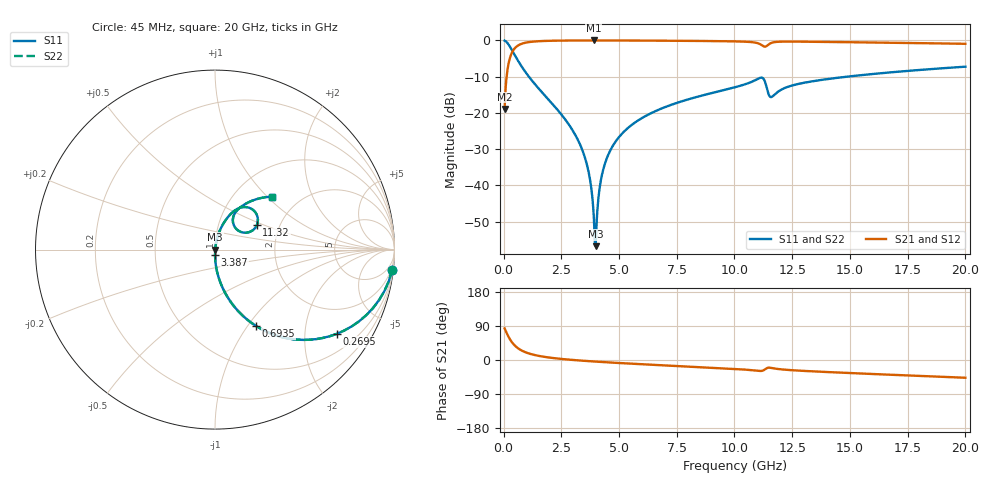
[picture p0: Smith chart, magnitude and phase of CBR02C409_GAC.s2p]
! S-parameter model data by Modelithics Inc.  support@modelithics.com 813-866-6335  Tampa FL USA
! S-Parameter data specifications:
! Substrate: 20-mil Rogers 4350B, substrate thickness, H=0.508mm, Dielectric constant, Er=3.75
! PCB Mounting Pad Footprint: Pad width, PadW=0.32mm , Pad length, PadL=0.37mm , Pad gap, PadG (edge-to-edge)=0.19mm , Reference planes=0.93mm apart
#  GHz  S  MA  R 50
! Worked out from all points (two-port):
!   801 points, 45 MHz to 20 GHz, reference 50 ohm
!   highest |S21| = -0.01 dB at 3.911 GHz (marker M1); lowest = -18.9 dB at 45 MHz (marker M2)
!   |S21| within 3 dB of the highest: 392 MHz to end of sweep
!   lowest |S11| = -56.8 dB at 3.986 GHz (marker M3), VSWR 1.00, Z = 50.1 + j0.0453 ohm
!   |S11| at or under -10 dB: 1.096 GHz to 14.88 GHz (13.78 GHz wide, 173 % of centre)
!   |S22| runs from -56.8 to -0.1 dB; largest |S21 - S12| = 0
!   S11 on the Smith chart (normalised r, x): 45 MHz: 1, -17; 269.5 MHz: 0.99, -2.90; 693.5 MHz: 0.99, -1.10; 3.387 GHz: 1.00, -0.06; 11.32 GHz: 1.53, +0.45; 20 GHz: 1.47, +1.07
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0.045  0.9936 -6.5  0.113 83.5  0.113 83.5  0.9936 -6.5
0.269494  0.825 -34.7  0.5646 55.3  0.5646 55.3  0.825 -34.7
0.693538  0.4837 -61.7  0.8744 28.2  0.8744 28.2  0.4837 -61.7
1.466794  0.2269 -78.2  0.9729 11.6  0.9729 11.6  0.2269 -78.2
2.738925  0.07579 -87.6  0.9959 1.5  0.9959 1.5  0.07579 -87.6
3.387462  0.03209 -89.4  0.9981 -1.7  0.9981 -1.7  0.03209 -89.4
3.711731  0.01378 -87.7  0.9985 -3.1  0.9985 -3.1  0.01378 -87.7
3.911281  0.003502 -71.5  0.9986 -3.9  0.9986 -3.9  0.003502 -71.5
3.986112  0.001451 18.1  0.9986 -4.2  0.9986 -4.2  0.001451 18.1
4.036  0.003326 61.7  0.9986 -4.4  0.9986 -4.4  0.003326 61.7
4.160719  0.009236 76.6  0.9985 -4.9  0.9985 -4.9  0.009236 76.6
4.260494  0.01396 79.1  0.9985 -5.3  0.9985 -5.3  0.01396 79.1
4.684538  0.03309 80.7  0.998 -6.8  0.998 -6.8  0.03309 80.7
5.457794  0.06474 79.2  0.9963 -9.5  0.9963 -9.5  0.06474 79.2
6.704981  0.1103 75.8  0.9922 -13.4  0.9922 -13.4  0.1103 75.8
10.0225  0.226 65.3  0.9696 -23.6  0.9696 -23.6  0.226 65.3
11.02025  0.2959 53.0  0.9126 -28.6  0.9126 -28.6  0.2959 53.0
11.31958  0.2697 30.2  0.82 -24.7  0.82 -24.7  0.2697 30.2
11.6189  0.1668 48.0  0.9284 -21.2  0.9284 -21.2  0.1668 48.0
13.36496  0.2727 59.2  0.9575 -29.9  0.9575 -29.9  0.2727 59.2
16.68248  0.3608 50.9  0.9297 -38.7  0.9297 -38.7  0.3608 50.9
20  0.434 42.8  0.898 -46.8  0.898 -46.8  0.434 42.8
